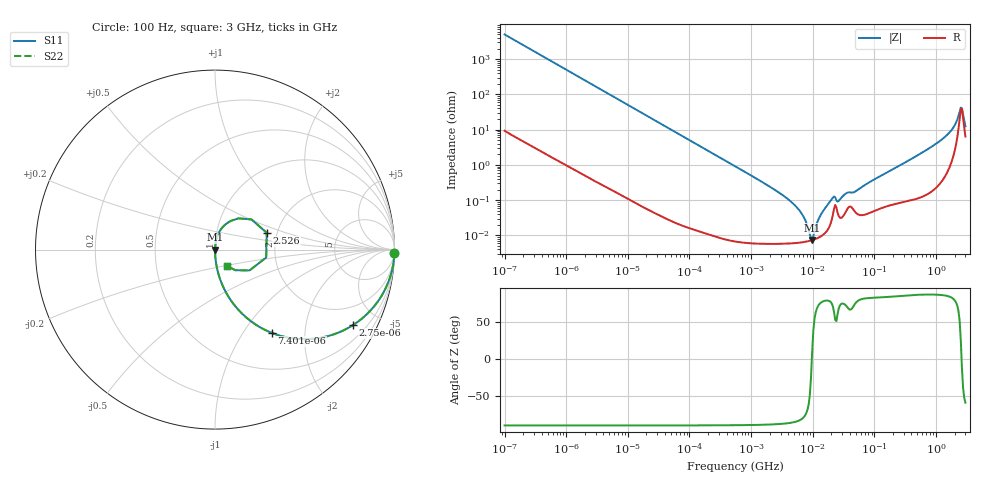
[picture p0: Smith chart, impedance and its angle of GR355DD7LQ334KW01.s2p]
!Murata Part Number: GR355DD7LQ334KW01
!These Parameters are Measured in Series Mode Connection
!Data Generated on Jun 19, 2026
!  o--ll--o
!Port1  Port2
!  o------o
!Operation Temp=25[degC], DC Bias Voltage=0[V]
!Freq. Start=100[Hz] Stop=3[GHz] 401[Steps]
# Hz S RI R 50
!Freq.(Hz) S11(Real) S11(Imag) S21(Real) S21(Imag) S12(Real) S12(Imag) S22(Real) S22(Imag)
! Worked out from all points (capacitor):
!   401 points, 100 Hz to 3 GHz, reference 50 ohm
!   read as one part in series: C = 318 nF near 109 Hz
!   lowest |Z| = 7.46 mohm at 9.794 MHz (marker M1)
!   series resonance near 9.674 MHz, so ESL is about 850 pH
!   S11 on the Smith chart (normalised r, x): 100 Hz: open; 2.75 kHz: 1.01, -3.65; 7.401 kHz: 1.00, -1.36; 2.526 GHz: 1.76, +0.36; 3 GHz: 1.13, -0.21
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100  0.9996 -0.02  0.000436 0.02  0.000436 0.02  0.9996 -0.02
536  0.9885 -0.1056  0.0115 0.1056  0.0115 0.1056  0.9885 -0.1056
1788  0.887 -0.3156  0.113 0.3156  0.113 0.3156  0.887 -0.3156
2750  0.769 -0.4204  0.231 0.4204  0.231 0.4204  0.769 -0.4204
7401  0.3164 -0.464  0.6836 0.464  0.6836 0.464  0.3164 -0.464
14115  0.1134 -0.316  0.8866 0.316  0.8866 0.316  0.1134 -0.316
31977  0.0246 -0.1537  0.9754 0.1537  0.9754 0.1537  0.0246 -0.1537
547723  0.000152 -0.00921  0.9998 0.00921  0.9998 0.00921  0.000152 -0.00921
4513443  6.02e-05 -0.000881  0.9999 0.000881  0.9999 0.000881  6.02e-05 -0.000881
6648799  6.37e-05 -0.000405  0.9999 0.000405  0.9999 0.000405  6.37e-05 -0.000405
8986547  7.04e-05 -7.84e-05  0.9999 7.84e-05  0.9999 7.84e-05  7.04e-05 -7.84e-05
9794414  7.34e-05 1.34e-05  0.9999 -1.34e-05  0.9999 -1.34e-05  7.34e-05 1.34e-05
1.382041e7  9.64e-05 0.000401  0.9999 -0.000401  0.9999 -0.000401  9.64e-05 0.000401
2.12544e7  0.000391 0.00111  0.9996 -0.00111  0.9996 -0.00111  0.000391 0.00111
2.635803e7  0.000359 0.000883  0.9996 -0.000883  0.9996 -0.000883  0.000359 0.000883
3.562563e7  0.000526 0.00151  0.9995 -0.00151  0.9995 -0.00151  0.000526 0.00151
4.815176e7  0.000479 0.00166  0.9995 -0.00166  0.9995 -0.00166  0.000479 0.00166
1.751444e8  0.000748 0.00659  0.9993 -0.00659  0.9993 -0.00659  0.000748 0.00659
1.268426e9  0.00646 0.0534  0.9935 -0.0534  0.9935 -0.0534  0.00646 0.0534
2.036508e9  0.0434 0.1263  0.9566 -0.1263  0.9566 -0.1263  0.0434 0.1263
2.525516e9  0.2882 0.0938  0.7118 -0.0938  0.7118 -0.0938  0.2882 0.0938
3e9  0.0692 -0.0931  0.9308 0.0931  0.9308 0.0931  0.0692 -0.0931
